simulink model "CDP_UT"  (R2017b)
settings: Solver=FixedStepDiscrete  StartTime=0.0  StopTime=10.0  FixedStep=0.01  RelTol=1e-3  EnableMultiTasking=on
undefined symbols (not defined in the file): ASWTYPE_FALSE, ASWTYPE_TRUE, CaCDP_CellTempNTCVoltTable_mV, CaCDP_CellTempTable_C, CaCDP_CMUPCBTempNTCVoltTable_mV, CaCDP_CMUPCBTempTable_C, CbCDP_DiffBusbarTempStateCheck_flg, CbCDP_DiffCellTempStateCheck_flg, CbCDP_DiffCellVoltStateCheck_flg, CbCDP_IgnorUpdateVld_flg, CbCDP_MaxBusbarTempStateCheck_flg, CbCDP_MaxCellTempStateCheck_flg, CbCDP_MaxCellVoltStateCheck_flg, CbCDP_MinBusbarTempStateCheck_flg, CbCDP_MinCellTempStateCheck_flg, CbCDP_MinCellVoltStateCheck_flg, CcCDP_AFETempConfig_numb, CcCDP_AFETempFltThd_C, CcCDP_AFETempFltThdHys_C, CcCDP_BusbarTempRngFltHiThrd_C, CcCDP_BusbarTempRngFltLowThrd_C, CcCDP_CellDiffFltLevel1_mV, CcCDP_CellDiffFltLevel2_mV, CcCDP_CellDiffFltLevel3_mV, CcCDP_CellTempLowerLimit_C, CcCDP_CellTempRngFltHiThrd_C, CcCDP_CellTempRngFltLowThrd_C, CcCDP_CellTempUpperLimit_C, CcCDP_CellVoltConfig_numb, CcCDP_CellVoltLowerLimit_mV, CcCDP_CellVoltRngHiThrd_mV, CcCDP_CellVoltRngLowThrd_mV, CcCDP_CellVoltUpdateThrd_numb, CcCDP_CellVoltUpperLimit_mV, CcCDP_ChrgMaxCellTempFltLv1Thrd_C, CcCDP_ChrgMaxCellTempFltLv2Thrd_C, CcCDP_ChrgMaxCellTempFltLv3Thrd_C, CcCDP_ChrgMaxCellTempReturnDiff_C, CcCDP_ChrgMinCellTempFltLv1Thrd_C, CcCDP_ChrgMinCellTempFltLv2Thrd_C, CcCDP_ChrgMinCellTempFltLv3Thrd_C, CcCDP_ChrgMinCellTempReturnDiff_C, CcCDP_CMUPCBTempConfig_numb, CcCDP_CMUPCBTempFltThd_C, CcCDP_CMUPCBTempFltThdHys_C, CcCDP_DiffBusbarTempFltLevel1Thrd_C, CcCDP_DiffBusbarTempFltLevel2Thrd_C, CcCDP_DiffBusbarTempReturnDifference_C, CcCDP_DiffCellTempFltLevel1Thrd_C, CcCDP_DiffCellTempFltLevel2Thrd_C, CcCDP_DiffCellTempReturnDifference_C, CcCDP_DiffCellVoltReturnDifference_mV, CcCDP_DiffVoltCheckMaxCellTempCondition_C, CcCDP_DiffVoltCheckMaxCellVoltCondition_mV, CcCDP_DiffVoltCheckMinCellTempCondition_C, CcCDP_DiffVoltCheckMinCellVoltCondition_mV, CcCDP_DiffVoltCheckPackCurrCondition_A, CcCDP_MaxAFETempIniVal_C, CcCDP_MaxBusbarTempFltLevel1Thrd_C, CcCDP_MaxBusbarTempFltLevel2Thrd_C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
libraries: AIWAYS_Powertrain_BMS_lib x148, simulink x8
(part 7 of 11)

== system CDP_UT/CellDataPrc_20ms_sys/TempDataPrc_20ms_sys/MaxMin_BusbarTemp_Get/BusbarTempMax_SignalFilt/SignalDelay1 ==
  u : Inport
  Bus to Vector : BusToVector
  Delay1Cycle : Subsystem
  Delay2Cycle : Subsystem
  Delay3Cycle : Subsystem
  Delay4Cycle : Subsystem
  Mux : Mux  Inputs=5
  y : Outport
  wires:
  u/1 -> Mux/1, Delay4Cycle/1(u), Delay3Cycle/1(u), Delay2Cycle/1(u), Delay1Cycle/1(u)
  Bus to Vector/1 -> y/1
  Delay4Cycle/1(y) -> Mux/5
  Delay2Cycle/1(y) -> Mux/3
  Delay3Cycle/1(y) -> Mux/4
  Delay1Cycle/1(y) -> Mux/2
  Mux/1 -> Bus to Vector/1

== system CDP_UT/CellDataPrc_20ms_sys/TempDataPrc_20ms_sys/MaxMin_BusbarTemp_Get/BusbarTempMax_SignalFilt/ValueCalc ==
  Output_Value : Inport
  Output_index : Inport  Port=2
  CcCDP_CellTempFilConfig_numb : Inport  Port=3
  Constant2 : Constant  Value=CDP_CONST1_NUMB
  Constant4 : Constant  Value=CDP_CONST2_NUMB
  Constant6 : Constant  Value=CDP_CONST1_NUMB
  Constant7 : Constant  Value=CDP_CONST2_NUMB
  Product1 : Product  Inputs=*/  OutDataTypeStr=Inherit: Inherit via back propagation
  Product2 : Product  Inputs=*/  OutDataTypeStr=Inherit: Inherit via back propagation
  Selector : Selector  InputPortWidth=5  IndexOptions=Index vector (port)  Indices=[1 3]  OutputSizes=1
  Selector1 : Selector  InputPortWidth=5  IndexOptions=Index vector (port)  Indices=[1 3]  OutputSizes=1
  Sum : Sum  OutDataTypeStr=Inherit: Inherit via back propagation  RndMeth=Zero
  Sum1 : Sum  OutDataTypeStr=Inherit: Inherit via back propagation  RndMeth=Zero
  GcCDP_MaxBusbarTemp_C : Outport
  Output_index1 : Outport  Port=2
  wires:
  Selector1/1 -> Output_index1/1
  Selector/1 -> GcCDP_MaxBusbarTemp_C/1
  Sum1/1 -> Product2/1
  Constant7/1 -> Product2/2
  Constant2/1 -> Sum/2
  Output_Value/1 -> Selector/1
  Constant6/1 -> Sum1/2
  Output_index/1 -> Selector1/1
  Sum/1 -> Product1/1
  Constant4/1 -> Product1/2
  Product1/1 -> Selector/2
  Product2/1 -> Selector1/2
  CcCDP_CellTempFilConfig_numb/1 -> Sum/1, Sum1/1

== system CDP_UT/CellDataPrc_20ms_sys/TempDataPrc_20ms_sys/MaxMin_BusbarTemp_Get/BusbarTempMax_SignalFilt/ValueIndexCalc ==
  Output_index1 : Inport
  LcCDP_MaxBusbarTempNumb_numb : Inport  Port=2
  LbCDP_AnyBusbarTempVld_flg : Inport  Port=3
  InputValueCalc1 : Stateflow chart  TreatAsAtomicUnit=on
  Selector2 : Selector  IndexMode=Zero-based  InputPortWidth=5  IndexOptions=Index vector (port)  Indices=[1 3]  OutputSizes=1
  Unit Delay1 : UnitDelay  SampleTime=-1  StateName=StateName
  GcCDP_MaxBusbarTempNumb_numb : Outport
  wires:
  LbCDP_AnyBusbarTempVld_flg/1 -> InputValueCalc1/2(Rige)
  Output_index1/1 -> Selector2/2
  InputValueCalc1/1(Output_Value) -> Selector2/1, Unit Delay1/1
  Unit Delay1/1 -> InputValueCalc1/3(Old_Value)
  LcCDP_MaxBusbarTempNumb_numb/1 -> InputValueCalc1/1(Input_Value)
  Selector2/1 -> GcCDP_MaxBusbarTempNumb_numb/1

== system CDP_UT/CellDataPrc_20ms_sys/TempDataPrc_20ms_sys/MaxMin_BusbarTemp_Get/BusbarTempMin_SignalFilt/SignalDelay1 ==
  u : Inport
  Bus to Vector : BusToVector
  Delay1Cycle : Subsystem
  Delay2Cycle : Subsystem
  Delay3Cycle : Subsystem
  Delay4Cycle : Subsystem
  Mux : Mux  Inputs=5
  y : Outport
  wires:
  Mux/1 -> Bus to Vector/1
  Delay1Cycle/1(y) -> Mux/2
  Delay3Cycle/1(y) -> Mux/4
  Delay2Cycle/1(y) -> Mux/3
  Delay4Cycle/1(y) -> Mux/5
  Bus to Vector/1 -> y/1
  u/1 -> Delay1Cycle/1(u), Delay2Cycle/1(u), Delay3Cycle/1(u), Delay4Cycle/1(u), Mux/1

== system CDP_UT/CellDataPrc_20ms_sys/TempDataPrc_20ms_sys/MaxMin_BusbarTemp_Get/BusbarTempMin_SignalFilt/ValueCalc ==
  Output_Value : Inport
  Output_index : Inport  Port=2
  CcCDP_CellTempFilConfig_numb : Inport  Port=3
  Constant2 : Constant  Value=CDP_CONST1_NUMB
  Constant4 : Constant  Value=CDP_CONST2_NUMB
  Constant6 : Constant  Value=CDP_CONST1_NUMB
  Constant7 : Constant  Value=CDP_CONST2_NUMB
  Product1 : Product  Inputs=*/  OutDataTypeStr=Inherit: Inherit via back propagation
  Product2 : Product  Inputs=*/  OutDataTypeStr=Inherit: Inherit via back propagation
  Selector : Selector  InputPortWidth=5  IndexOptions=Index vector (port)  Indices=[1 3]  OutputSizes=1
  Selector1 : Selector  InputPortWidth=5  IndexOptions=Index vector (port)  Indices=[1 3]  OutputSizes=1
  Sum : Sum  OutDataTypeStr=Inherit: Inherit via back propagation  RndMeth=Zero
  Sum1 : Sum  OutDataTypeStr=Inherit: Inherit via back propagation  RndMeth=Zero
  GcCDP_MinBusbarTemp_C : Outport
  Output_index1 : Outport  Port=2
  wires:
  CcCDP_CellTempFilConfig_numb/1 -> Sum1/1, Sum/1
  Product2/1 -> Selector1/2
  Product1/1 -> Selector/2
  Constant4/1 -> Product1/2
  Sum/1 -> Product1/1
  Output_index/1 -> Selector1/1
  Constant6/1 -> Sum1/2
  Output_Value/1 -> Selector/1
  Constant2/1 -> Sum/2
  Constant7/1 -> Product2/2
  Sum1/1 -> Product2/1
  Selector/1 -> GcCDP_MinBusbarTemp_C/1
  Selector1/1 -> Output_index1/1

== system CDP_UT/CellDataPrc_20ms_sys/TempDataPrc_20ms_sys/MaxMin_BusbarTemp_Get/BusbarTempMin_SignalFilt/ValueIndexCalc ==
  Output_index1 : Inport
  LcCDP_MinBusbarTempNumb_numb : Inport  Port=2
  LbCDP_AnyBusbarTempVld_flg : Inport  Port=3
  InputValueCalc1 : Stateflow chart  TreatAsAtomicUnit=on
  Selector2 : Selector  IndexMode=Zero-based  InputPortWidth=5  IndexOptions=Index vector (port)  Indices=[1 3]  OutputSizes=1
  Unit Delay1 : UnitDelay  SampleTime=-1  StateName=StateName
  GcCDP_MinBusbarTempNumb_numb : Outport
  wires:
  Selector2/1 -> GcCDP_MinBusbarTempNumb_numb/1
  LcCDP_MinBusbarTempNumb_numb/1 -> InputValueCalc1/1(Input_Value)
  Unit Delay1/1 -> InputValueCalc1/3(Old_Value)
  InputValueCalc1/1(Output_Value) -> Unit Delay1/1, Selector2/1
  Output_index1/1 -> Selector2/2
  LbCDP_AnyBusbarTempVld_flg/1 -> InputValueCalc1/2(Rige)

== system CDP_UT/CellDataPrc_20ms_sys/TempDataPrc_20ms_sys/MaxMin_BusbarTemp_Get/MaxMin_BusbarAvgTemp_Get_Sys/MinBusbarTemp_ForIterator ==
  LaCDP_BusbarTemp_C : Inport
  GcUDS_BusbarTempNumb_numb : Inport  Port=2
  Add : Sum  AccumDataTypeStr=single  OutDataTypeStr=single
  MinBusbarTempNumbIterator : ForIterator  ResetStates=reset  IterationSource=external  IterationVariableDataType=int8
  Selector1 : Selector  IndexOptions=Index vector (port)  Indices=[1 3]  OutputSizes=1
  Unit Delay : UnitDelay  SampleTime=-1  StateName=StateName
  LcCDP_SumBusbarTemp_C : Outport
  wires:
  Selector1/1 -> Add/2  "LcCDP_IniOutputSumBusbarTemp_C"
  Unit Delay/1 -> Add/1
  LaCDP_BusbarTemp_C/1 -> Selector1/1
  MinBusbarTempNumbIterator/1 -> Selector1/2
  GcUDS_BusbarTempNumb_numb/1 -> MinBusbarTempNumbIterator/1
  Add/1 -> Unit Delay/1, LcCDP_SumBusbarTemp_C/1  "LcCDP_SumBusbarTemp_C"

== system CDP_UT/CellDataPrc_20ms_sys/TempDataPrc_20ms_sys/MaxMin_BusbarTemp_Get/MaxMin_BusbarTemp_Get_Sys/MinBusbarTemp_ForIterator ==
  LaCDP_BusbarTemp_C : Inport
  LaCDP_BusbarTempVld_flg : Inport  Port=2
  GcUDS_BusbarTempNumb_numb : Inport  Port=3
  Bus Creator : BusCreator  Inputs=3
  Bus Selector : BusSelector  OutputSignals=LcCDP_IniOutputBusbarTemp_C,LcCDP_IniOutputBusbarTempNumb_numb,LbCDP_IniOutputBusbarTempVld_flg
  Bus Selector1 : BusSelector  OutputSignals=LcCDP_IniOutputBusbarTemp_C,LcCDP_IniOutputBusbarTempNumb_numb,LbCDP_IniOutputBusbarTempVld_flg
  Data Type Conversion : DataTypeConversion
  MaxBusbarTemp_ForIterator : Subsystem
  MinBusbarTempNumbIterator : ForIterator  ResetStates=reset  IterationSource=external  IterationVariableDataType=int8
  MinBusbarTemp_ForIterator : Subsystem
  Selector1 : Selector  IndexOptions=Index vector (port)  Indices=[1 3]  OutputSizes=1
  Selector2 : Selector  IndexOptions=Index vector (port)  Indices=[1 3]  OutputSizes=1
  LcCDP_MinBusbarTemp_C : Outport
  LcCDP_MinBusbarTempNumb_numb : Outport  Port=2
  LcCDP_MaxBusbarTempNumb_numb : Outport  Port=3
  LcCDP_MaxBusbarTemp_C : Outport  Port=4
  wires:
  Bus Selector1/3 -> MaxBusbarTemp_ForIterator/3(LbCDP_IniOutputBusbarTempVld_flg)  "<LbCDP_IniOutputBusbarTempVld_flg>"
  Bus Selector/3 -> MinBusbarTemp_ForIterator/3(LbCDP_IniOutputBusbarTempVld_flg)  "<LbCDP_IniOutputBusbarTempVld_flg>"
  Selector2/1 -> Bus Creator/3  "LbCDP_IniOutputBusbarTempVld_flg"
  LaCDP_BusbarTempVld_flg/1 -> Selector2/1
  MaxBusbarTemp_ForIterator/1(LcCDP_MaxBusbarTempNumb_numb) -> LcCDP_MaxBusbarTempNumb_numb/1
  MaxBusbarTemp_ForIterator/2(LcCDP_MaxBusbarTemp_C) -> LcCDP_MaxBusbarTemp_C/1
  MinBusbarTemp_ForIterator/2(LcCDP_MinBusbarTempNumb_numb) -> LcCDP_MinBusbarTempNumb_numb/1
  MinBusbarTemp_ForIterator/1(LcCDP_MinBusbarTemp_C) -> LcCDP_MinBusbarTemp_C/1
  Bus Creator/1 -> Bus Selector/1, Bus Selector1/1
  GcUDS_BusbarTempNumb_numb/1 -> MinBusbarTempNumbIterator/1
  MinBusbarTempNumbIterator/1 -> Selector1/2, Data Type Conversion/1, Selector2/2
  LaCDP_BusbarTemp_C/1 -> Selector1/1
  Selector1/1 -> Bus Creator/1  "LcCDP_IniOutputBusbarTemp_C"
  Data Type Conversion/1 -> Bus Creator/2  "LcCDP_IniOutputBusbarTempNumb_numb"
  Bus Selector/1 -> MinBusbarTemp_ForIterator/1(LcCDP_IniOutputBusbarTemp_C)  "<LcCDP_IniOutputBusbarTemp_C>"
  Bus Selector/2 -> MinBusbarTemp_ForIterator/2(LcCDP_IniOutputBusbarTempNumb_numb)  "<LcCDP_IniOutputBusbarTempNumb_numb>"
  Bus Selector1/1 -> MaxBusbarTemp_ForIterator/1(LcCDP_IniOutputBusbarTemp_C)  "<LcCDP_IniOutputBusbarTemp_C>"
  Bus Selector1/2 -> MaxBusbarTemp_ForIterator/2(LcCDP_IniOutputBusbarTempNumb_numb)  "<LcCDP_IniOutputBusbarTempNumb_numb>"

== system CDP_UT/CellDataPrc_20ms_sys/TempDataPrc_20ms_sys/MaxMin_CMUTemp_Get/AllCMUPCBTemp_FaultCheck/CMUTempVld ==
  GaCDP_CMUPCBTempVld_flg : Inport
  CcCDP_CMUTempConfig_numb : Inport  Port=2
  CMUTemp : ForIterator  ResetStates=reset  IterationSource=external  IterationVariableDataType=int16
  Logical Operator1 : Logic  Operator=OR  AllPortsSameDT=off  OutDataTypeStr=boolean
  Selector : Selector  IndexOptions=Index vector (port)  Indices=[1 3]  OutputSizes=1
  Unit Delay1 : UnitDelay  SampleTime=-1  StateName=StateName
  LbCDP_AnyCMUTempVld_flg : Outport
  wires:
  Selector/1 -> Logical Operator1/2
  CMUTemp/1 -> Selector/2
  CcCDP_CMUTempConfig_numb/1 -> CMUTemp/1
  GaCDP_CMUPCBTempVld_flg/1 -> Selector/1
  Logical Operator1/1 -> Unit Delay1/1, LbCDP_AnyCMUTempVld_flg/1  "LbCDP_AnyCMUTempVld_flg"
  Unit Delay1/1 -> Logical Operator1/1

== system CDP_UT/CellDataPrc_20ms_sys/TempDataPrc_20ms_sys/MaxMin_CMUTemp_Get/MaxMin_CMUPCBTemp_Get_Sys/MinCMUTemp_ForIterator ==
  GaCDP_CMUPCBTemp_C : Inport
  GaCDP_CMUPCBTempVld_flg : Inport  Port=2
  CcCDP_CMUPCBTempConfig_numb : Inport  Port=3
  Bus Creator : BusCreator  Inputs=3
  Bus Selector : BusSelector  OutputSignals=LcCDP_IniOutputCMUPCBTemp_C,LcCDP_IniOutputCMUPCBTempNumb_numb,LbCDP_IniOutputCMUPCBTempVld_flg
  Bus Selector1 : BusSelector  OutputSignals=LcCDP_IniOutputCMUPCBTemp_C,LcCDP_IniOutputCMUPCBTempNumb_numb,LbCDP_IniOutputCMUPCBTempVld_flg
  Data Type Conversion : DataTypeConversion
  MaxCMUTemp_ForIterator : Subsystem
  MinCMUTempNumbIterator : ForIterator  ResetStates=reset  IterationSource=external  IterationVariableDataType=int8
  MinCMUTemp_ForIterator : Subsystem
  Selector1 : Selector  IndexOptions=Index vector (port)  Indices=[1 3]  OutputSizes=1
  Selector2 : Selector  IndexOptions=Index vector (port)  Indices=[1 3]  OutputSizes=1
  LcCDP_MinCMUPCBTemp_C : Outport
  LcCDP_MinCMUPCBTempNumb_numb : Outport  Port=2
  LcCDP_MaxCMUPCBTempNumb_numb : Outport  Port=3
  LcCDP_MaxCMUPCBTemp_C : Outport  Port=4
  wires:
  Bus Selector1/2 -> MaxCMUTemp_ForIterator/2(LcCDP_IniOutputCMUPCBTempNumb_numb)  "<LcCDP_IniOutputCMUPCBTempNumb_numb>"
  Bus Selector1/1 -> MaxCMUTemp_ForIterator/1(LcCDP_IniOutputCMUPCBTemp_C)  "<LcCDP_IniOutputCMUPCBTemp_C>"
  Bus Selector/2 -> MinCMUTemp_ForIterator/2(LcCDP_IniOutputCMUPCBTempNumb_numb)  "<LcCDP_IniOutputCMUPCBTempNumb_numb>"
  Bus Selector/1 -> MinCMUTemp_ForIterator/1(LcCDP_IniOutputCMUPCBTemp_C)  "<LcCDP_IniOutputCMUPCBTemp_C>"
  Data Type Conversion/1 -> Bus Creator/2  "LcCDP_IniOutputCMUPCBTempNumb_numb"
  Selector1/1 -> Bus Creator/1  "LcCDP_IniOutputCMUPCBTemp_C"
  GaCDP_CMUPCBTemp_C/1 -> Selector1/1
  MinCMUTempNumbIterator/1 -> Selector2/2, Data Type Conversion/1, Selector1/2
  CcCDP_CMUPCBTempConfig_numb/1 -> MinCMUTempNumbIterator/1
  Bus Creator/1 -> Bus Selector/1, Bus Selector1/1
  MinCMUTemp_ForIterator/1(LcCDP_MinCMUPCBTemp_C) -> LcCDP_MinCMUPCBTemp_C/1
  MinCMUTemp_ForIterator/2(LcCDP_MinCMUPCBTempNumb_numb) -> LcCDP_MinCMUPCBTempNumb_numb/1
  MaxCMUTemp_ForIterator/2(LcCDP_MaxCMUPCBTemp_C) -> LcCDP_MaxCMUPCBTemp_C/1
  MaxCMUTemp_ForIterator/1(LcCDP_MaxCMUPCBTempNumb_numb) -> LcCDP_MaxCMUPCBTempNumb_numb/1
  GaCDP_CMUPCBTempVld_flg/1 -> Selector2/1
  Selector2/1 -> Bus Creator/3  "LbCDP_IniOutputCMUPCBTempVld_flg"
  Bus Selector/3 -> MinCMUTemp_ForIterator/3(LbCDP_IniOutputCMUPCBTempVld_flg)  "<LbCDP_IniOutputCMUPCBTempVld_flg>"
  Bus Selector1/3 -> MaxCMUTemp_ForIterator/3(LbCDP_IniOutputCMUPCBTempVld_flg)  "<LbCDP_IniOutputCMUPCBTempVld_flg>"

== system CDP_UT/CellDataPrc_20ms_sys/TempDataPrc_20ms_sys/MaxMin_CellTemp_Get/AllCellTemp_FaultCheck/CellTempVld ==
  GaCDP_CellTempVld_flg : Inport
  GcUDS_CellTempNumb_numb : Inport  Port=2
  CellTemp : ForIterator  ResetStates=reset  IterationSource=external  IterationVariableDataType=int16
  Logical Operator : Logic  AllPortsSameDT=off  OutDataTypeStr=boolean
  Logical Operator1 : Logic  Operator=OR  AllPortsSameDT=off  OutDataTypeStr=boolean
  Selector : Selector  IndexOptions=Index vector (port)  Indices=[1 3]  OutputSizes=1
  Unit Delay : UnitDelay  InitialCondition=ASWTYPE_TRUE  SampleTime=-1  StateName=StateName
  Unit Delay1 : UnitDelay  SampleTime=-1  StateName=StateName
  LbCDP_CellTempVld_flg : Outport
  LbCDP_AnyCellTempVld_flg : Outport  Port=2
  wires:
  Selector/1 -> Logical Operator/1, Logical Operator1/2
  CellTemp/1 -> Selector/2
  GcUDS_CellTempNumb_numb/1 -> CellTemp/1
  Logical Operator/1 -> Unit Delay/1, LbCDP_CellTempVld_flg/1
  GaCDP_CellTempVld_flg/1 -> Selector/1
  Unit Delay/1 -> Logical Operator/2
  Logical Operator1/1 -> Unit Delay1/1, LbCDP_AnyCellTempVld_flg/1  "LbCDP_AnyCellTempVld_flg"
  Unit Delay1/1 -> Logical Operator1/1

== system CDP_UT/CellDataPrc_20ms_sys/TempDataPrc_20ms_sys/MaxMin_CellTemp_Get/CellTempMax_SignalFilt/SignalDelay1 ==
  u : Inport
  Bus to Vector : BusToVector
  Delay1Cycle : Subsystem
  Delay2Cycle : Subsystem
  Delay3Cycle : Subsystem
  Delay4Cycle : Subsystem
  Mux : Mux  Inputs=5
  y : Outport
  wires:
  u/1 -> Mux/1, Delay4Cycle/1(u), Delay3Cycle/1(u), Delay2Cycle/1(u), Delay1Cycle/1(u)
  Bus to Vector/1 -> y/1
  Delay4Cycle/1(y) -> Mux/5
  Delay2Cycle/1(y) -> Mux/3
  Delay3Cycle/1(y) -> Mux/4
  Delay1Cycle/1(y) -> Mux/2
  Mux/1 -> Bus to Vector/1

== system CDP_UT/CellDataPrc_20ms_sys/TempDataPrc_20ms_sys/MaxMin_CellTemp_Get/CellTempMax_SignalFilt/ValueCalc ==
  Output_Value : Inport
  Output_index : Inport  Port=2
  CcCDP_CellTempFilConfig_numb : Inport  Port=3
  Constant2 : Constant  Value=CDP_CONST1_NUMB
  Constant4 : Constant  Value=CDP_CONST2_NUMB
  Constant6 : Constant  Value=CDP_CONST1_NUMB
  Constant7 : Constant  Value=CDP_CONST2_NUMB
  Product1 : Product  Inputs=*/  OutDataTypeStr=Inherit: Inherit via back propagation
  Product2 : Product  Inputs=*/  OutDataTypeStr=Inherit: Inherit via back propagation
  Selector : Selector  InputPortWidth=5  IndexOptions=Index vector (port)  Indices=[1 3]  OutputSizes=1
  Selector1 : Selector  InputPortWidth=5  IndexOptions=Index vector (port)  Indices=[1 3]  OutputSizes=1
  Sum : Sum  OutDataTypeStr=Inherit: Inherit via back propagation  RndMeth=Zero
  Sum1 : Sum  OutDataTypeStr=Inherit: Inherit via back propagation  RndMeth=Zero
  GcCDP_MaxCellTemp_C : Outport
  Output_index1 : Outport  Port=2
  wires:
  Selector1/1 -> Output_index1/1
  Selector/1 -> GcCDP_MaxCellTemp_C/1
  Sum1/1 -> Product2/1
  Constant7/1 -> Product2/2
  Constant2/1 -> Sum/2
  Output_Value/1 -> Selector/1
  Constant6/1 -> Sum1/2
  Output_index/1 -> Selector1/1
  Sum/1 -> Product1/1
  Constant4/1 -> Product1/2
  Product1/1 -> Selector/2
  Product2/1 -> Selector1/2
  CcCDP_CellTempFilConfig_numb/1 -> Sum/1, Sum1/1

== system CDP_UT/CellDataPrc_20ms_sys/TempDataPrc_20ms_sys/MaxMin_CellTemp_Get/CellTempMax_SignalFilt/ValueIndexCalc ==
  Output_index1 : Inport
  LcCDP_MaxCellTempNumb_numb : Inport  Port=2
  LbCDP_AnyCellTempVld_flg : Inport  Port=3
  InputValueCalc1 : Stateflow chart  TreatAsAtomicUnit=on
  Selector2 : Selector  IndexMode=Zero-based  InputPortWidth=5  IndexOptions=Index vector (port)  Indices=[1 3]  OutputSizes=1
  Unit Delay1 : UnitDelay  SampleTime=-1  StateName=StateName
  GcCDP_MaxCellTempNumb_numb : Outport
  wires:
  LbCDP_AnyCellTempVld_flg/1 -> InputValueCalc1/2(Rige)
  Output_index1/1 -> Selector2/2
  InputValueCalc1/1(Output_Value) -> Selector2/1, Unit Delay1/1
  Unit Delay1/1 -> InputValueCalc1/3(Old_Value)
  LcCDP_MaxCellTempNumb_numb/1 -> InputValueCalc1/1(Input_Value)
  Selector2/1 -> GcCDP_MaxCellTempNumb_numb/1

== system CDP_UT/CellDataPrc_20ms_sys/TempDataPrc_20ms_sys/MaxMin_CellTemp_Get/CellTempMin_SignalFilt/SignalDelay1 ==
  u : Inport
  Bus to Vector : BusToVector
  Delay1Cycle : Subsystem
  Delay2Cycle : Subsystem
  Delay3Cycle : Subsystem
  Delay4Cycle : Subsystem
  Mux : Mux  Inputs=5
  y : Outport
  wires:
  Mux/1 -> Bus to Vector/1
  Delay1Cycle/1(y) -> Mux/2
  Delay3Cycle/1(y) -> Mux/4
  Delay2Cycle/1(y) -> Mux/3
  Delay4Cycle/1(y) -> Mux/5
  Bus to Vector/1 -> y/1
  u/1 -> Delay1Cycle/1(u), Delay2Cycle/1(u), Delay3Cycle/1(u), Delay4Cycle/1(u), Mux/1

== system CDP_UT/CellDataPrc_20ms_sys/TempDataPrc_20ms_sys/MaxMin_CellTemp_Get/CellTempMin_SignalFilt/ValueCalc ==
  Output_Value : Inport
  Output_index : Inport  Port=2
  CcCDP_CellTempFilConfig_numb : Inport  Port=3
  Constant2 : Constant  Value=CDP_CONST1_NUMB
  Constant4 : Constant  Value=CDP_CONST2_NUMB
  Constant6 : Constant  Value=CDP_CONST1_NUMB
  Constant7 : Constant  Value=CDP_CONST2_NUMB
  Product1 : Product  Inputs=*/  OutDataTypeStr=Inherit: Inherit via back propagation
  Product2 : Product  Inputs=*/  OutDataTypeStr=Inherit: Inherit via back propagation
  Selector : Selector  InputPortWidth=5  IndexOptions=Index vector (port)  Indices=[1 3]  OutputSizes=1
  Selector1 : Selector  InputPortWidth=5  IndexOptions=Index vector (port)  Indices=[1 3]  OutputSizes=1
  Sum : Sum  OutDataTypeStr=Inherit: Inherit via back propagation  RndMeth=Zero
  Sum1 : Sum  OutDataTypeStr=Inherit: Inherit via back propagation  RndMeth=Zero
  GcCDP_MinCellTemp_C : Outport
  Output_index1 : Outport  Port=2
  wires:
  CcCDP_CellTempFilConfig_numb/1 -> Sum1/1, Sum/1
  Product2/1 -> Selector1/2
  Product1/1 -> Selector/2
  Constant4/1 -> Product1/2
  Sum/1 -> Product1/1
  Output_index/1 -> Selector1/1
  Constant6/1 -> Sum1/2
  Output_Value/1 -> Selector/1
  Constant2/1 -> Sum/2
  Constant7/1 -> Product2/2
  Sum1/1 -> Product2/1
  Selector/1 -> GcCDP_MinCellTemp_C/1
  Selector1/1 -> Output_index1/1

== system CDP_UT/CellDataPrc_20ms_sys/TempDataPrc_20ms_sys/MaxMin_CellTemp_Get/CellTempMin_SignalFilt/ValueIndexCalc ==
  Output_index1 : Inport
  LcCDP_MinCellTempNumb_numb : Inport  Port=2
  LbCDP_AnyCellTempVld_flg : Inport  Port=3
  InputValueCalc1 : Stateflow chart  TreatAsAtomicUnit=on
  Selector2 : Selector  IndexMode=Zero-based  InputPortWidth=5  IndexOptions=Index vector (port)  Indices=[1 3]  OutputSizes=1
  Unit Delay1 : UnitDelay  SampleTime=-1  StateName=StateName
  GcCDP_MinCellTempNumb_numb : Outport
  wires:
  Selector2/1 -> GcCDP_MinCellTempNumb_numb/1
  LcCDP_MinCellTempNumb_numb/1 -> InputValueCalc1/1(Input_Value)
  Unit Delay1/1 -> InputValueCalc1/3(Old_Value)
  InputValueCalc1/1(Output_Value) -> Unit Delay1/1, Selector2/1
  Output_index1/1 -> Selector2/2
  LbCDP_AnyCellTempVld_flg/1 -> InputValueCalc1/2(Rige)

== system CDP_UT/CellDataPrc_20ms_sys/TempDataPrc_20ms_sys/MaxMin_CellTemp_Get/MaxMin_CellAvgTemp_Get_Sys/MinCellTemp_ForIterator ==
  LaCDP_CellTemp_C : Inport
  GcUDS_CellTempNumb_numb : Inport  Port=2
  Add : Sum  AccumDataTypeStr=single  OutDataTypeStr=single
  MinCellTempNumbIterator : ForIterator  ResetStates=reset  IterationSource=external  IterationVariableDataType=int8
  Selector1 : Selector  IndexOptions=Index vector (port)  Indices=[1 3]  OutputSizes=1
  Unit Delay : UnitDelay  SampleTime=-1  StateName=StateName
  LcCDP_SumCellTemp_C : Outport
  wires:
  Add/1 -> LcCDP_SumCellTemp_C/1, Unit Delay/1  "LcCDP_SumCellTemp_C"
  GcUDS_CellTempNumb_numb/1 -> MinCellTempNumbIterator/1
  MinCellTempNumbIterator/1 -> Selector1/2
  LaCDP_CellTemp_C/1 -> Selector1/1
  Unit Delay/1 -> Add/1
  Selector1/1 -> Add/2  "LcCDP_IniOutputSumCellTemp_C"

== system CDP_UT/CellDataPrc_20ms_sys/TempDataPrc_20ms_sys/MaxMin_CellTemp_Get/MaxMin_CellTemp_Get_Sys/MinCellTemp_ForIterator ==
  LaCDP_CellTemp_C : Inport
  GaCDP_CellTempVld_flg : Inport  Port=2
  GcUDS_CellTempNumb_numb : Inport  Port=3
  Bus Creator : BusCreator  Inputs=3
  Bus Selector : BusSelector  OutputSignals=LcCDP_IniOutputCellTemp_C,LcCDP_IniOutputCellTempNumb_numb,LbCDP_IniOutputCellTempVld_flg
  Bus Selector1 : BusSelector  OutputSignals=LcCDP_IniOutputCellTemp_C,LcCDP_IniOutputCellTempNumb_numb,LbCDP_IniOutputCellTempVld_flg
  Data Type Conversion : DataTypeConversion
  MaxCellTemp_ForIterator : Subsystem
  MinCellTempNumbIterator : ForIterator  ResetStates=reset  IterationSource=external  IterationVariableDataType=int8
  MinCellTemp_ForIterator : Subsystem
  Selector1 : Selector  IndexOptions=Index vector (port)  Indices=[1 3]  OutputSizes=1
  Selector2 : Selector  IndexOptions=Index vector (port)  Indices=[1 3]  OutputSizes=1
  LcCDP_MinCellTemp_C : Outport
  LcCDP_MinCellTempNumb_numb : Outport  Port=2
  LcCDP_MaxCellTempNumb_numb : Outport  Port=3
  LcCDP_MaxCellTemp_C : Outport  Port=4
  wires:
  Bus Selector1/2 -> MaxCellTemp_ForIterator/2(LcCDP_IniOutputCellTempNumb_numb)  "<LcCDP_IniOutputCellTempNumb_numb>"
  Bus Selector1/1 -> MaxCellTemp_ForIterator/1(LcCDP_IniOutputCellTemp_C)  "<LcCDP_IniOutputCellTemp_C>"
  Bus Selector/2 -> MinCellTemp_ForIterator/2(LcCDP_IniOutputCellTempNumb_numb)  "<LcCDP_IniOutputCellTempNumb_numb>"
  Bus Selector/1 -> MinCellTemp_ForIterator/1(LcCDP_IniOutputCellTemp_C)  "<LcCDP_IniOutputCellTemp_C>"
  Data Type Conversion/1 -> Bus Creator/2  "LcCDP_IniOutputCellTempNumb_numb"
  Selector1/1 -> Bus Creator/1  "LcCDP_IniOutputCellTemp_C"
  LaCDP_CellTemp_C/1 -> Selector1/1
  MinCellTempNumbIterator/1 -> Selector2/2, Data Type Conversion/1, Selector1/2
  GcUDS_CellTempNumb_numb/1 -> MinCellTempNumbIterator/1
  Bus Creator/1 -> Bus Selector1/1, Bus Selector/1
  MinCellTemp_ForIterator/1(LcCDP_MinCellTemp_C) -> LcCDP_MinCellTemp_C/1
  MinCellTemp_ForIterator/2(LcCDP_MinCellTempNumb_numb) -> LcCDP_MinCellTempNumb_numb/1
  MaxCellTemp_ForIterator/2(LcCDP_MaxCellTemp_C) -> LcCDP_MaxCellTemp_C/1
  MaxCellTemp_ForIterator/1(LcCDP_MaxCellTempNumb_numb) -> LcCDP_MaxCellTempNumb_numb/1
  GaCDP_CellTempVld_flg/1 -> Selector2/1
  Selector2/1 -> Bus Creator/3  "LbCDP_IniOutputCellTempVld_flg"
  Bus Selector/3 -> MinCellTemp_ForIterator/3(LbCDP_IniOutputCellTempVld_flg)  "<LbCDP_IniOutputCellTempVld_flg>"
  Bus Selector1/3 -> MaxCellTemp_ForIterator/3(LbCDP_IniOutputCellTempVld_flg)  "<LbCDP_IniOutputCellTempVld_flg>"

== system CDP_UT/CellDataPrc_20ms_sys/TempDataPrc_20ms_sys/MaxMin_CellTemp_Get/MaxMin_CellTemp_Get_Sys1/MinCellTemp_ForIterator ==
  GaCDP_CellTemp_C : Inport
  GaCDP_CellTempVld_flg : Inport  Port=2
  GcUDS_CellTempNumb_numb : Inport  Port=3
  Bus Creator : BusCreator  Inputs=3
  Bus Selector : BusSelector  OutputSignals=LcCDP_IniOutputCellTemp_C,LcCDP_IniOutputCellTempNumb_numb,LbCDP_IniOutputCellTempVld_flg
  Bus Selector1 : BusSelector  OutputSignals=LcCDP_IniOutputCellTemp_C,LcCDP_IniOutputCellTempNumb_numb,LbCDP_IniOutputCellTempVld_flg
  Data Type Conversion : DataTypeConversion
  MaxCellTemp_ForIterator : Subsystem
  MinCellTempNumbIterator : ForIterator  ResetStates=reset  IterationSource=external  IterationVariableDataType=int8
  MinCellTemp_ForIterator : Subsystem
  Selector1 : Selector  IndexOptions=Index vector (port)  Indices=[1 3]  OutputSizes=1
  Selector2 : Selector  IndexOptions=Index vector (port)  Indices=[1 3]  OutputSizes=1
  LcCDP_MinCellTemp_C : Outport
  LcCDP_MinCellTempNumb_numb : Outport  Port=2
  LcCDP_MaxCellTempNumb_numb : Outport  Port=3
  LcCDP_MaxCellTemp_C : Outport  Port=4
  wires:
  Bus Selector1/2 -> MaxCellTemp_ForIterator/2(LcCDP_IniOutputCellTempNumb_numb)  "<LcCDP_IniOutputCellTempNumb_numb>"
  Bus Selector1/1 -> MaxCellTemp_ForIterator/1(LcCDP_IniOutputCellTemp_C)  "<LcCDP_IniOutputCellTemp_C>"
  Bus Selector/2 -> MinCellTemp_ForIterator/2(LcCDP_IniOutputCellTempNumb_numb)  "<LcCDP_IniOutputCellTempNumb_numb>"
  Bus Selector/1 -> MinCellTemp_ForIterator/1(LcCDP_IniOutputCellTemp_C)  "<LcCDP_IniOutputCellTemp_C>"
  Data Type Conversion/1 -> Bus Creator/2  "LcCDP_IniOutputCellTempNumb_numb"
  Selector1/1 -> Bus Creator/1  "LcCDP_IniOutputCellTemp_C"
  GaCDP_CellTemp_C/1 -> Selector1/1
  MinCellTempNumbIterator/1 -> Selector2/2, Data Type Conversion/1, Selector1/2
  GcUDS_CellTempNumb_numb/1 -> MinCellTempNumbIterator/1
  Bus Creator/1 -> Bus Selector1/1, Bus Selector/1
  MinCellTemp_ForIterator/1(LcCDP_MinCellTemp_C) -> LcCDP_MinCellTemp_C/1
  MinCellTemp_ForIterator/2(LcCDP_MinCellTempNumb_numb) -> LcCDP_MinCellTempNumb_numb/1
  MaxCellTemp_ForIterator/2(LcCDP_MaxCellTemp_C) -> LcCDP_MaxCellTemp_C/1
  MaxCellTemp_ForIterator/1(LcCDP_MaxCellTempNumb_numb) -> LcCDP_MaxCellTempNumb_numb/1
  GaCDP_CellTempVld_flg/1 -> Selector2/1
  Selector2/1 -> Bus Creator/3  "LbCDP_IniOutputCellTempVld_flg"
  Bus Selector/3 -> MinCellTemp_ForIterator/3(LbCDP_IniOutputCellTempVld_flg)  "<LbCDP_IniOutputCellTempVld_flg>"
  Bus Selector1/3 -> MaxCellTemp_ForIterator/3(LbCDP_IniOutputCellTempVld_flg)  "<LbCDP_IniOutputCellTempVld_flg>"

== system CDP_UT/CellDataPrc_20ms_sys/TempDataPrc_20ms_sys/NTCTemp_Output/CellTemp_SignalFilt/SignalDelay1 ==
  u : Inport
  Bus to Vector : BusToVector
  Delay1Cycle : Subsystem
  Delay2Cycle : Subsystem
  Delay3Cycle : Subsystem
  Delay4Cycle : Subsystem
  Mux : Mux  Inputs=5
  y : Outport
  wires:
  u/1 -> Mux/1, Delay4Cycle/1(u), Delay3Cycle/1(u), Delay2Cycle/1(u), Delay1Cycle/1(u)
  Bus to Vector/1 -> y/1
  Delay4Cycle/1(y) -> Mux/5
  Delay2Cycle/1(y) -> Mux/3
  Delay3Cycle/1(y) -> Mux/4
  Delay1Cycle/1(y) -> Mux/2
  Mux/1 -> Bus to Vector/1

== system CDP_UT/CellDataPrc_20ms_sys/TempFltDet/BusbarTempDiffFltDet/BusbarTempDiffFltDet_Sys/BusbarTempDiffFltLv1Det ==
  LbCDP_DiffBusbarTempChkCond_flg : Inport
  LcCDP_DiffBusbarTemp_C : Inport  Port=2
  LbCDP_BusbarTempRngHiFlt_flg : Inport  Port=3
  LbCDP_BusbarTempRngLowFlt_flg : Inport  Port=4
  Add4 : Sum  OutDataTypeStr=Inherit: Inherit via back propagation
  CDP_GbCDP_ChrgMaxCellVoltFltLv1_flg : AIWAYS_Powertrain_BMS_lib/Signals/OverWrite  OverWrite_Value=CbCDP_BusbarTempDiffFltLv1Ovr_flg  OverWrite_flag=CbCDP_BusbarTempDiffFltLv1OvrSwt_flg
  Constant : Constant  Value=CcCDP_DiffBusbarTempFltLevel1Thrd_C
  Constant1 : Constant  Value=ASWTYPE_FALSE
  Constant2 : Constant  Value=CcCDP_DiffBusbarTempReturnDifference_C
  Constant3 : Constant  Value=ASWTYPE_FALSE
  Constant4 : Constant  Value=ASWTYPE_TRUE
  Constant7 : Constant  Value=ASWTYPE_TRUE
  Logical Operator : Logic  Inputs=4  AllPortsSameDT=off  OutDataTypeStr=boolean
  Logical Operator1 : Logic  AllPortsSameDT=off  OutDataTypeStr=boolean
  Relational Operator : RelationalOperator  OutDataTypeStr=boolean
  Relational Operator1 : RelationalOperator  Operator===  OutDataTypeStr=boolean
  Relational Operator2 : RelationalOperator  Operator===  OutDataTypeStr=boolean
  Relational Operator3 : RelationalOperator  Operator===  OutDataTypeStr=boolean
  GbCDP_BusbarTempDiffFltLv1_flg : Outport
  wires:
  Constant7/1 -> Logical Operator1/1
  Logical Operator1/1 -> Logical Operator/1
  LcCDP_DiffBusbarTemp_C/1 -> Relational Operator/1
  Relational Operator3/1 -> Logical Operator/4
  Constant4/1 -> Relational Operator3/2
  LbCDP_DiffBusbarTempChkCond_flg/1 -> Relational Operator3/1
  Relational Operator2/1 -> Logical Operator/3
  Constant3/1 -> Relational Operator2/2
  LbCDP_BusbarTempRngLowFlt_flg/1 -> Relational Operator2/1
  LbCDP_BusbarTempRngHiFlt_flg/1 -> Relational Operator1/1
  Logical Operator/1 -> CDP_GbCDP_ChrgMaxCellVoltFltLv1_flg/1
  Relational Operator/1 -> Logical Operator1/2
  Constant1/1 -> Relational Operator1/2
  Relational Operator1/1 -> Logical Operator/2
  Constant/1 -> Add4/1
  CDP_GbCDP_ChrgMaxCellVoltFltLv1_flg/1 -> GbCDP_BusbarTempDiffFltLv1_flg/1  "GbCDP_BusbarTempDiffFltLv1_flg"
  Constant2/1 -> Add4/2
  Add4/1 -> Relational Operator/2

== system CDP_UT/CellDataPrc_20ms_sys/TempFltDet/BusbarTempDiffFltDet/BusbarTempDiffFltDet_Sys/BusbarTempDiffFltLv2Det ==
  LcCDP_DiffBusbarTemp_C : Inport
  LbCDP_BusbarTempRngHiFlt_flg : Inport  Port=2
  LbCDP_BusbarTempRngLowFlt_flg : Inport  Port=3
  LbCDP_DiffBusbarTempChkCond_flg : Inport  Port=4
  Add4 : Sum  OutDataTypeStr=Inherit: Inherit via back propagation
  CDP_GbCDP_ChrgMaxCellVoltFltLv1_flg : AIWAYS_Powertrain_BMS_lib/Signals/OverWrite  OverWrite_Value=CbCDP_BusbarTempDiffFltLv2Ovr_flg  OverWrite_flag=CbCDP_BusbarTempDiffFltLv2OvrSwt_flg
  Constant : Constant  Value=CcCDP_DiffBusbarTempFltLevel2Thrd_C
  Constant1 : Constant  Value=ASWTYPE_FALSE
  Constant2 : Constant  Value=CcCDP_DiffBusbarTempReturnDifference_C
  Constant3 : Constant  Value=ASWTYPE_FALSE
  Constant4 : Constant  Value=ASWTYPE_TRUE
  Logical Operator : Logic  Inputs=4  AllPortsSameDT=off  OutDataTypeStr=boolean
  Relational Operator : RelationalOperator  OutDataTypeStr=boolean
  Relational Operator1 : RelationalOperator  Operator===  OutDataTypeStr=boolean
  Relational Operator2 : RelationalOperator  Operator===  OutDataTypeStr=boolean
  Relational Operator3 : RelationalOperator  Operator===  OutDataTypeStr=boolean
  GbCDP_BusbarTempDiffFltLv2_flg : Outport
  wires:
  Relational Operator3/1 -> Logical Operator/4
  Constant4/1 -> Relational Operator3/2
  LbCDP_DiffBusbarTempChkCond_flg/1 -> Relational Operator3/1
  Add4/1 -> Relational Operator/2
  Constant2/1 -> Add4/2
  LcCDP_DiffBusbarTemp_C/1 -> Relational Operator/1
  CDP_GbCDP_ChrgMaxCellVoltFltLv1_flg/1 -> GbCDP_BusbarTempDiffFltLv2_flg/1  "GbCDP_BusbarTempDiffFltLv2_flg"
  Constant/1 -> Add4/1
  Relational Operator1/1 -> Logical Operator/2
  Constant1/1 -> Relational Operator1/2
  Relational Operator/1 -> Logical Operator/1
  Logical Operator/1 -> CDP_GbCDP_ChrgMaxCellVoltFltLv1_flg/1
  LbCDP_BusbarTempRngHiFlt_flg/1 -> Relational Operator1/1
  LbCDP_BusbarTempRngLowFlt_flg/1 -> Relational Operator2/1
  Constant3/1 -> Relational Operator2/2
  Relational Operator2/1 -> Logical Operator/3

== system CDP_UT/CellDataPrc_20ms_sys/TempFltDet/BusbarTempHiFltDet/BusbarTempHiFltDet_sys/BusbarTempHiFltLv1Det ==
  LbCDP_MaxBusbarTempChkCond_flg : Inport
  GcCDP_MaxBusbarTemp_C : Inport  Port=2
  Add4 : Sum  OutDataTypeStr=Inherit: Inherit via back propagation
  CDP_GbCDP_ChrgMaxCellVoltFltLv1_flg : AIWAYS_Powertrain_BMS_lib/Signals/OverWrite  OverWrite_Value=CbCDP_BusbarTempHiFltLv1Ovr_flg  OverWrite_flag=CbCDP_BusbarTempHiFltLv1OvrSwt_flg
  Constant : Constant  Value=CcCDP_MaxBusbarTempFltLevel1Thrd_C
  Constant1 : Constant  Value=ASWTYPE_TRUE
  Constant2 : Constant  Value=CcCDP_MaxBusbarTempReturnDifference_C
  Constant4 : Constant  Value=ASWTYPE_TRUE
  Logical Operator : Logic  AllPortsSameDT=off  OutDataTypeStr=boolean
  Logical Operator1 : Logic  AllPortsSameDT=off  OutDataTypeStr=boolean
  Relational Operator : RelationalOperator  OutDataTypeStr=boolean
  Relational Operator1 : RelationalOperator  Operator===  OutDataTypeStr=boolean
  GbCDP_BusbarTempHiFltLv1_flg : Outport
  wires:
  Logical Operator/1 -> CDP_GbCDP_ChrgMaxCellVoltFltLv1_flg/1
  CDP_GbCDP_ChrgMaxCellVoltFltLv1_flg/1 -> GbCDP_BusbarTempHiFltLv1_flg/1  "GbCDP_BusbarTempHiFltLv1_flg"
  Logical Operator1/1 -> Logical Operator/1
  Relational Operator/1 -> Logical Operator1/2
  Constant/1 -> Add4/1
  Relational Operator1/1 -> Logical Operator/2
  Constant2/1 -> Add4/2
  Add4/1 -> Relational Operator/2
  LbCDP_MaxBusbarTempChkCond_flg/1 -> Relational Operator1/1
  Constant1/1 -> Relational Operator1/2
  GcCDP_MaxBusbarTemp_C/1 -> Relational Operator/1
  Constant4/1 -> Logical Operator1/1

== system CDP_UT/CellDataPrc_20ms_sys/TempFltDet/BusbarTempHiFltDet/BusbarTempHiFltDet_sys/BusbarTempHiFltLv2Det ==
  LbCDP_MaxBusbarTempChkCond_flg : Inport
  GcCDP_MaxBusbarTemp_C : Inport  Port=2
  Add4 : Sum  OutDataTypeStr=Inherit: Inherit via back propagation
  CDP_GbCDP_ChrgMaxCellVoltFltLv1_flg : AIWAYS_Powertrain_BMS_lib/Signals/OverWrite  OverWrite_Value=CbCDP_BusbarTempHiFltLv2Ovr_flg  OverWrite_flag=CbCDP_BusbarTempHiFltLv2OvrSwt_flg
  Constant : Constant  Value=CcCDP_MaxBusbarTempFltLevel2Thrd_C
  Constant1 : Constant  Value=ASWTYPE_TRUE
  Constant2 : Constant  Value=CcCDP_MaxBusbarTempReturnDifference_C
  Constant4 : Constant  Value=ASWTYPE_TRUE
  Logical Operator : Logic  AllPortsSameDT=off  OutDataTypeStr=boolean
  Logical Operator1 : Logic  AllPortsSameDT=off  OutDataTypeStr=boolean
  Relational Operator : RelationalOperator  OutDataTypeStr=boolean
  Relational Operator1 : RelationalOperator  Operator===  OutDataTypeStr=boolean
  GbCDP_BusbarTempHiFltLv2_flg : Outport
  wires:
  Constant4/1 -> Logical Operator1/1
  GcCDP_MaxBusbarTemp_C/1 -> Relational Operator/1
  Constant1/1 -> Relational Operator1/2
  LbCDP_MaxBusbarTempChkCond_flg/1 -> Relational Operator1/1
  Add4/1 -> Relational Operator/2
  Constant2/1 -> Add4/2
  Relational Operator1/1 -> Logical Operator/2
  Constant/1 -> Add4/1
  Relational Operator/1 -> Logical Operator1/2
  Logical Operator1/1 -> Logical Operator/1
  CDP_GbCDP_ChrgMaxCellVoltFltLv1_flg/1 -> GbCDP_BusbarTempHiFltLv2_flg/1  "GbCDP_BusbarTempHiFltLv2_flg"
  Logical Operator/1 -> CDP_GbCDP_ChrgMaxCellVoltFltLv1_flg/1

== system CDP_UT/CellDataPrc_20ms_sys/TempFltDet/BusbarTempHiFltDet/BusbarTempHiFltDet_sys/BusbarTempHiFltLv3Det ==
  LbCDP_MaxBusbarTempChkCond_flg : Inport
  GcCDP_MaxBusbarTemp_C : Inport  Port=2
  Add4 : Sum  OutDataTypeStr=Inherit: Inherit via back propagation
  CDP_GbCDP_ChrgMaxCellVoltFltLv1_flg : AIWAYS_Powertrain_BMS_lib/Signals/OverWrite  OverWrite_Value=CbCDP_BusbarTempHiFltLv3Ovr_flg  OverWrite_flag=CbCDP_BusbarTempHiFltLv3OvrSwt_flg
  Comparison : RelationalOperator  Operator=>  OutDataTypeStr=boolean
  Constant : Constant  Value=CcCDP_MaxBusbarTempFltLevel3Thrd_C
  Constant1 : Constant  Value=ASWTYPE_TRUE
  Constant2 : Constant  Value=CcCDP_MaxBusbarTempReturnDifference_C
  Constant3 : Constant  Value=CcCDP_BusbarTempRngFltHiThrd_C
  Constant4 : Constant  Value=ASWTYPE_TRUE
  Logical Operator : Logic  AllPortsSameDT=off  OutDataTypeStr=boolean
  Logical Operator1 : Logic  AllPortsSameDT=off  OutDataTypeStr=boolean
  Relational Operator : RelationalOperator  OutDataTypeStr=boolean
  Relational Operator1 : RelationalOperator  Operator===  OutDataTypeStr=boolean
  Terminator : Terminator
  GbCDP_BusbarTempHiFltLv3_flg : Outport
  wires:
  Logical Operator/1 -> CDP_GbCDP_ChrgMaxCellVoltFltLv1_flg/1
  CDP_GbCDP_ChrgMaxCellVoltFltLv1_flg/1 -> GbCDP_BusbarTempHiFltLv3_flg/1  "GbCDP_BusbarTempHiFltLv3_flg"
  Logical Operator1/1 -> Logical Operator/1
  Comparison/1 -> Terminator/1
  Relational Operator/1 -> Logical Operator1/2
  Constant/1 -> Add4/1
  Relational Operator1/1 -> Logical Operator/2
  Constant2/1 -> Add4/2
  Add4/1 -> Relational Operator/2
  LbCDP_MaxBusbarTempChkCond_flg/1 -> Relational Operator1/1
  Constant1/1 -> Relational Operator1/2
  GcCDP_MaxBusbarTemp_C/1 -> Relational Operator/1, Comparison/2
  Constant3/1 -> Comparison/1
  Constant4/1 -> Logical Operator1/1

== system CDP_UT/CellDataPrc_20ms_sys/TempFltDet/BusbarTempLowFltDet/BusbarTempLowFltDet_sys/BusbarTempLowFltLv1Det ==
  LbCDP_MinBusbarTempChkCond_flg : Inport
  GcCDP_MinBusbarTemp_C : Inport  Port=2
  Add4 : Sum  OutDataTypeStr=Inherit: Inherit via back propagation
  CDP_GbCDP_ChrgMaxCellVoltFltLv1_flg : AIWAYS_Powertrain_BMS_lib/Signals/OverWrite  OverWrite_Value=CbCDP_BusbarTempLowFltLv1Ovr_flg  OverWrite_flag=CbCDP_BusbarTempLowFltLv1OvrSwt_flg
  Constant : Constant  Value=CcCDP_MinBusbarTempFltLevel1Thrd_C
  Constant1 : Constant  Value=ASWTYPE_TRUE
  Constant2 : Constant  Value=CcCDP_MinBusbarTempReturnDifference_C
  Constant4 : Constant  Value=ASWTYPE_TRUE
  Logical Operator : Logic  AllPortsSameDT=off  OutDataTypeStr=boolean
  Logical Operator1 : Logic  AllPortsSameDT=off  OutDataTypeStr=boolean
  Relational Operator1 : RelationalOperator  Operator===  OutDataTypeStr=boolean
  Relational Operator3 : RelationalOperator  Operator=<=  OutDataTypeStr=boolean
  GbCDP_BusbarTempLowFltLv1_flg : Outport
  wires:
  Logical Operator/1 -> CDP_GbCDP_ChrgMaxCellVoltFltLv1_flg/1
  CDP_GbCDP_ChrgMaxCellVoltFltLv1_flg/1 -> GbCDP_BusbarTempLowFltLv1_flg/1  "GbCDP_BusbarTempLowFltLv1_flg"
  Logical Operator1/1 -> Logical Operator/1
  Relational Operator3/1 -> Logical Operator1/2
  Constant/1 -> Add4/1
  Relational Operator1/1 -> Logical Operator/2
  Constant2/1 -> Add4/2
  Add4/1 -> Relational Operator3/2
  LbCDP_MinBusbarTempChkCond_flg/1 -> Relational Operator1/1
  Constant1/1 -> Relational Operator1/2
  GcCDP_MinBusbarTemp_C/1 -> Relational Operator3/1
  Constant4/1 -> Logical Operator1/1

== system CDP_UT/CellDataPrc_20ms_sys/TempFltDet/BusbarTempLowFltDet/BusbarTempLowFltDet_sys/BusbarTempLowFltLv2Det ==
  LbCDP_MinBusbarTempChkCond_flg : Inport
  GcCDP_MinBusbarTemp_C : Inport  Port=2
  Add4 : Sum  OutDataTypeStr=Inherit: Inherit via back propagation
  CDP_GbCDP_ChrgMaxCellVoltFltLv1_flg : AIWAYS_Powertrain_BMS_lib/Signals/OverWrite  OverWrite_Value=CbCDP_BusbarTempLowFltLv2Ovr_flg  OverWrite_flag=CbCDP_BusbarTempLowFltLv2OvrSwt_flg
  Constant : Constant  Value=CcCDP_MinBusbarTempFltLevel2Thrd_C
  Constant1 : Constant  Value=ASWTYPE_TRUE
  Constant2 : Constant  Value=CcCDP_MinBusbarTempReturnDifference_C
  Constant4 : Constant  Value=ASWTYPE_TRUE
  Logical Operator : Logic  AllPortsSameDT=off  OutDataTypeStr=boolean
  Logical Operator1 : Logic  AllPortsSameDT=off  OutDataTypeStr=boolean
  Relational Operator1 : RelationalOperator  Operator===  OutDataTypeStr=boolean
  Relational Operator3 : RelationalOperator  Operator=<=  OutDataTypeStr=boolean
  GbCDP_BusbarTempLowFltLv2_flg : Outport
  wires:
  Constant4/1 -> Logical Operator1/1
  GcCDP_MinBusbarTemp_C/1 -> Relational Operator3/1
  Constant1/1 -> Relational Operator1/2
  LbCDP_MinBusbarTempChkCond_flg/1 -> Relational Operator1/1
  Add4/1 -> Relational Operator3/2
  Constant2/1 -> Add4/2
  Relational Operator1/1 -> Logical Operator/2
  Constant/1 -> Add4/1
  Relational Operator3/1 -> Logical Operator1/2
  Logical Operator1/1 -> Logical Operator/1
  CDP_GbCDP_ChrgMaxCellVoltFltLv1_flg/1 -> GbCDP_BusbarTempLowFltLv2_flg/1  "GbCDP_BusbarTempLowFltLv2_flg"
  Logical Operator/1 -> CDP_GbCDP_ChrgMaxCellVoltFltLv1_flg/1

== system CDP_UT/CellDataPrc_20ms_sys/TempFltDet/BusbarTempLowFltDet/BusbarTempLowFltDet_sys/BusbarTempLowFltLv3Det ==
  LbCDP_MinBusbarTempChkCond_flg : Inport
  GcCDP_MinBusbarTemp_C : Inport  Port=2
  Add4 : Sum  OutDataTypeStr=Inherit: Inherit via back propagation
  CDP_GbCDP_ChrgMaxCellVoltFltLv1_flg : AIWAYS_Powertrain_BMS_lib/Signals/OverWrite  OverWrite_Value=CbCDP_BusbarTempLowFltLv3Ovr_flg  OverWrite_flag=CbCDP_BusbarTempLowFltLv3OvrSwt_flg
  Comparison1 : RelationalOperator  Operator=<  OutDataTypeStr=boolean
  Constant : Constant  Value=CcCDP_MinBusbarTempFltLevel3Thrd_C
  Constant1 : Constant  Value=ASWTYPE_TRUE
  Constant2 : Constant  Value=CcCDP_MinBusbarTempReturnDifference_C
  Constant3 : Constant  Value=CcCDP_BusbarTempRngFltLowThrd_C
  Constant4 : Constant  Value=ASWTYPE_TRUE
  Logical Operator : Logic  AllPortsSameDT=off  OutDataTypeStr=boolean
  Logical Operator1 : Logic  AllPortsSameDT=off  OutDataTypeStr=boolean
  Relational Operator1 : RelationalOperator  Operator===  OutDataTypeStr=boolean
  Relational Operator3 : RelationalOperator  Operator=<=  OutDataTypeStr=boolean
  Terminator : Terminator
  GbCDP_BusbarTempLowFltLv3_flg : Outport
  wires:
  Logical Operator/1 -> CDP_GbCDP_ChrgMaxCellVoltFltLv1_flg/1
  CDP_GbCDP_ChrgMaxCellVoltFltLv1_flg/1 -> GbCDP_BusbarTempLowFltLv3_flg/1  "GbCDP_BusbarTempLowFltLv3_flg"
  Logical Operator1/1 -> Logical Operator/1
  Comparison1/1 -> Terminator/1
  Relational Operator3/1 -> Logical Operator1/2
  Constant/1 -> Add4/1
  Relational Operator1/1 -> Logical Operator/2
  Constant2/1 -> Add4/2
  Add4/1 -> Relational Operator3/2
  LbCDP_MinBusbarTempChkCond_flg/1 -> Relational Operator1/1
  Constant1/1 -> Relational Operator1/2
  GcCDP_MinBusbarTemp_C/1 -> Relational Operator3/1, Comparison1/2
  Constant3/1 -> Comparison1/1
  Constant4/1 -> Logical Operator1/1

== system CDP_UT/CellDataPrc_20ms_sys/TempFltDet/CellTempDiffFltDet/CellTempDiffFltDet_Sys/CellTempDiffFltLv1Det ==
  LbCDP_DiffTempCheckCondition_flg : Inport
  LcCDP_DiffCellTemp_C : Inport  Port=2
  LbCDP_CellTempRngHiFlt_flg : Inport  Port=3
  LbCDP_CellTempRngLowFlt_flg : Inport  Port=4
  Add1 : Sum  OutDataTypeStr=Inherit: Inherit via back propagation
  Add4 : Sum  OutDataTypeStr=Inherit: Inherit via back propagation
  CDP_GbCDP_ChrgMaxCellVoltFltLv1_flg : AIWAYS_Powertrain_BMS_lib/Signals/OverWrite  OverWrite_Value=CbCDP_CellTempDiffFltLv1Ovr_flg  OverWrite_flag=CbCDP_CellTempDiffFltLv1OvrSwt_flg
  Comparison : RelationalOperator  Operator=>  OutDataTypeStr=boolean
  Constant : Constant  Value=CcCDP_DiffCellTempFltLevel1Thrd_C
  Constant1 : Constant  Value=ASWTYPE_FALSE
  Constant2 : Constant  Value=CcCDP_DiffCellTempReturnDifference_C
  Constant3 : Constant  Value=ASWTYPE_FALSE
  Constant4 : Constant  Value=ASWTYPE_TRUE
  Constant5 : Constant  Value=CcCDP_DiffCellTempFltLevel2Thrd_C
  Constant6 : Constant  Value=CcCDP_DiffCellTempReturnDifference_C
  Constant7 : Constant  Value=ASWTYPE_TRUE
  Logical Operator : Logic  Inputs=4  AllPortsSameDT=off  OutDataTypeStr=boolean
  Logical Operator1 : Logic  AllPortsSameDT=off  OutDataTypeStr=boolean
  Relational Operator : RelationalOperator  OutDataTypeStr=boolean
  Relational Operator1 : RelationalOperator  Operator===  OutDataTypeStr=boolean
  Relational Operator2 : RelationalOperator  Operator===  OutDataTypeStr=boolean
  Relational Operator3 : RelationalOperator  Operator===  OutDataTypeStr=boolean
  Terminator : Terminator
  GbCDP_CellTempDiffFltLv1_flg : Outport
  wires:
  Add4/1 -> Relational Operator/2
  Constant2/1 -> Add4/2
  CDP_GbCDP_ChrgMaxCellVoltFltLv1_flg/1 -> GbCDP_CellTempDiffFltLv1_flg/1  "GbCDP_CellTempDiffFltLv1_flg"
  Constant/1 -> Add4/1
  Relational Operator1/1 -> Logical Operator/2
  Constant1/1 -> Relational Operator1/2
  Relational Operator/1 -> Logical Operator1/2
  Logical Operator/1 -> CDP_GbCDP_ChrgMaxCellVoltFltLv1_flg/1
  LbCDP_CellTempRngHiFlt_flg/1 -> Relational Operator1/1
  LbCDP_CellTempRngLowFlt_flg/1 -> Relational Operator2/1
  Constant3/1 -> Relational Operator2/2
  Relational Operator2/1 -> Logical Operator/3
  LbCDP_DiffTempCheckCondition_flg/1 -> Relational Operator3/1
  Constant4/1 -> Relational Operator3/2
  Relational Operator3/1 -> Logical Operator/4
  LcCDP_DiffCellTemp_C/1 -> Relational Operator/1, Comparison/2
  Constant5/1 -> Add1/1
  Constant6/1 -> Add1/2
  Add1/1 -> Comparison/1
  Comparison/1 -> Terminator/1
  Logical Operator1/1 -> Logical Operator/1
  Constant7/1 -> Logical Operator1/1

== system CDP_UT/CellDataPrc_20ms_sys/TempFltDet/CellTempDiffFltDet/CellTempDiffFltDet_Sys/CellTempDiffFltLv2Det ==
  LcCDP_DiffCellTemp_C : Inport
  LbCDP_CellTempRngHiFlt_flg : Inport  Port=2
  LbCDP_CellTempRngLowFlt_flg : Inport  Port=3
  LbCDP_DiffTempCheckCondition_flg : Inport  Port=4
  Add4 : Sum  OutDataTypeStr=Inherit: Inherit via back propagation
  CDP_GbCDP_ChrgMaxCellVoltFltLv1_flg : AIWAYS_Powertrain_BMS_lib/Signals/OverWrite  OverWrite_Value=CbCDP_CellTempDiffFltLv2Ovr_flg  OverWrite_flag=CbCDP_CellTempDiffFltLv2OvrSwt_flg
  Constant : Constant  Value=CcCDP_DiffCellTempFltLevel2Thrd_C
  Constant1 : Constant  Value=ASWTYPE_FALSE
  Constant2 : Constant  Value=CcCDP_DiffCellTempReturnDifference_C
  Constant3 : Constant  Value=ASWTYPE_FALSE
  Constant4 : Constant  Value=ASWTYPE_TRUE
  Logical Operator : Logic  Inputs=4  AllPortsSameDT=off  OutDataTypeStr=boolean
  Relational Operator : RelationalOperator  OutDataTypeStr=boolean
  Relational Operator1 : RelationalOperator  Operator===  OutDataTypeStr=boolean
  Relational Operator2 : RelationalOperator  Operator===  OutDataTypeStr=boolean
  Relational Operator3 : RelationalOperator  Operator===  OutDataTypeStr=boolean
  GbCDP_CellTempDiffFltLv2_flg : Outport
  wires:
  Relational Operator2/1 -> Logical Operator/3
  Constant3/1 -> Relational Operator2/2
  LbCDP_CellTempRngLowFlt_flg/1 -> Relational Operator2/1
  LbCDP_CellTempRngHiFlt_flg/1 -> Relational Operator1/1
  Logical Operator/1 -> CDP_GbCDP_ChrgMaxCellVoltFltLv1_flg/1
  Relational Operator/1 -> Logical Operator/1
  Constant1/1 -> Relational Operator1/2
  Relational Operator1/1 -> Logical Operator/2
  Constant/1 -> Add4/1
  CDP_GbCDP_ChrgMaxCellVoltFltLv1_flg/1 -> GbCDP_CellTempDiffFltLv2_flg/1  "GbCDP_CellTempDiffFltLv2_flg"
  LcCDP_DiffCellTemp_C/1 -> Relational Operator/1
  Constant2/1 -> Add4/2
  Add4/1 -> Relational Operator/2
  LbCDP_DiffTempCheckCondition_flg/1 -> Relational Operator3/1
  Constant4/1 -> Relational Operator3/2
  Relational Operator3/1 -> Logical Operator/4

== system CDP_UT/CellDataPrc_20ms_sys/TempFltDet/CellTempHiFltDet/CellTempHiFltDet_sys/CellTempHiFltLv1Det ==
  LbCDP_MaxTempCheckCondition_flg : Inport
  GcCDP_MaxCellTemp_C : Inport  Port=2
  Add1 : Sum  OutDataTypeStr=Inherit: Inherit via back propagation
  Add4 : Sum  OutDataTypeStr=Inherit: Inherit via back propagation
  CDP_GbCDP_ChrgMaxCellVoltFltLv1_flg : AIWAYS_Powertrain_BMS_lib/Signals/OverWrite  OverWrite_Value=CbCDP_CellTempHiFltLv1Ovr_flg  OverWrite_flag=CbCDP_CellTempHiFltLv1OvrSwt_flg
  Comparison : RelationalOperator  Operator=>  OutDataTypeStr=boolean
  Constant : Constant  Value=CcCDP_MaxCellTempFltLevel1Thrd_C
  Constant1 : Constant  Value=ASWTYPE_TRUE
  Constant2 : Constant  Value=CcCDP_MaxCellTempReturnDifference_C
  Constant3 : Constant  Value=CcCDP_MaxCellTempFltLevel2Thrd_C
  Constant4 : Constant  Value=CcCDP_MaxCellTempReturnDifference_C
  Constant5 : Constant  Value=ASWTYPE_TRUE
  Logical Operator : Logic  AllPortsSameDT=off  OutDataTypeStr=boolean
  Logical Operator1 : Logic  AllPortsSameDT=off  OutDataTypeStr=boolean
  Relational Operator : RelationalOperator  OutDataTypeStr=boolean
  Relational Operator1 : RelationalOperator  Operator===  OutDataTypeStr=boolean
  Terminator : Terminator
  GbCDP_CellTempHiFltLv1_flg : Outport
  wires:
  Logical Operator/1 -> CDP_GbCDP_ChrgMaxCellVoltFltLv1_flg/1
  CDP_GbCDP_ChrgMaxCellVoltFltLv1_flg/1 -> GbCDP_CellTempHiFltLv1_flg/1  "GbCDP_CellTempHiFltLv1_flg"
  Logical Operator1/1 -> Logical Operator/1
  Add1/1 -> Comparison/1
  Comparison/1 -> Terminator/1
  Constant3/1 -> Add1/1
  Relational Operator/1 -> Logical Operator1/2
  Constant/1 -> Add4/1
  Relational Operator1/1 -> Logical Operator/2
  Constant2/1 -> Add4/2
  Add4/1 -> Relational Operator/2
  Constant4/1 -> Add1/2
  LbCDP_MaxTempCheckCondition_flg/1 -> Relational Operator1/1
  Constant1/1 -> Relational Operator1/2
  GcCDP_MaxCellTemp_C/1 -> Relational Operator/1, Comparison/2
  Constant5/1 -> Logical Operator1/1
